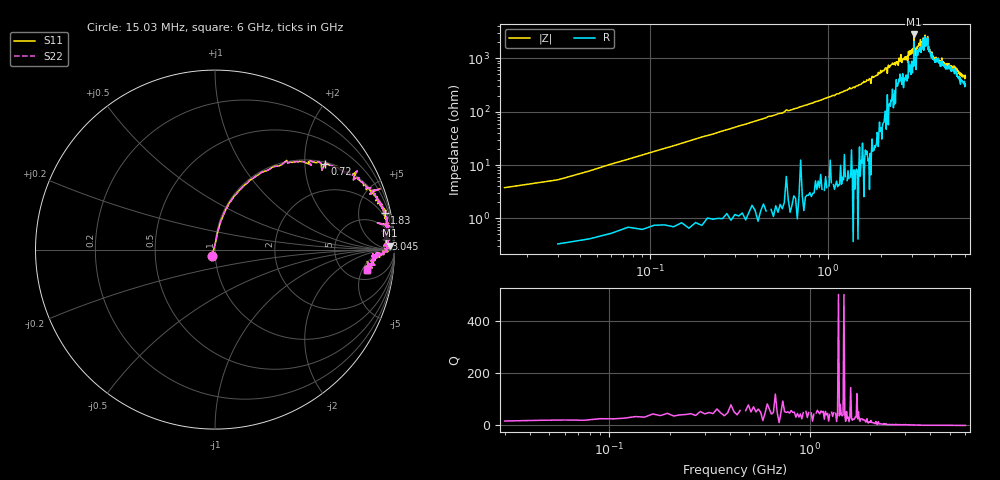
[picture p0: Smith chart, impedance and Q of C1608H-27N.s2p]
!	Network	Analyzer	HP8753E.07.74:	Oct	30	2002	Serial	No.	JP38451487
!	Hewlett-Packard
!	7	Sep	2009	10:22:24
!	Frequency	S11	S21	S12	S22
#	HZ	S	RI	R	50
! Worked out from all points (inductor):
!   400 points, 15.03 MHz to 6 GHz, reference 50 ohm
!   read as one part in series: L = 27.3 nH near 45.03 MHz
!   highest |Z| = 2.79 kohm at 3.075 GHz (marker M1)
!   self-resonance near 3.52 GHz
!   S11 on the Smith chart (normalised r, x): 15.03 MHz: 0.97, -0.07; 720 MHz: 1.05, +2.52; 1.83 GHz: 1.38, +9.08; 3.045 GHz: 15, +20; 6 GHz: 7.37, -6.16
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1.502992e7  -0.0162 -0.0339  1.02 0.0339  1.02 0.0339  -0.0162 -0.0339
9.002955e7  0.0291 0.149  0.971 -0.149  0.971 -0.149  0.0291 0.149
1.95029e8  0.106 0.297  0.894 -0.297  0.894 -0.297  0.106 0.297
7.200264e8  0.612 0.477  0.388 -0.477  0.388 -0.477  0.612 0.477
1.020025e9  0.775 0.407  0.225 -0.407  0.225 -0.407  0.775 0.407
1.830021e9  0.946 0.206  0.054 -0.206  0.054 -0.206  0.946 0.206
2.01002e9  0.952 0.172  0.0476 -0.172  0.0476 -0.172  0.952 0.172
2.595017e9  0.964 0.0741  0.0365 -0.0741  0.0365 -0.0741  0.964 0.0741
2.835016e9  0.936 0.0912  0.0645 -0.0912  0.0645 -0.0912  0.936 0.0912
2.865016e9  0.951 0.051  0.049 -0.051  0.049 -0.051  0.951 0.051
3.015015e9  0.973 0.0591  0.0266 -0.0591  0.0266 -0.0591  0.973 0.0591
3.045015e9  0.951 0.0602  0.0494 -0.0602  0.0494 -0.0602  0.951 0.0602
3.075015e9  0.973 0.0225  0.0266 -0.0225  0.0266 -0.0225  0.973 0.0225
3.090015e9  0.956 0.0476  0.044 -0.0476  0.044 -0.0476  0.956 0.0476
3.165014e9  0.947 0.0681  0.0529 -0.0681  0.0529 -0.0681  0.947 0.0681
3.555012e9  0.966 0.0113  0.0337 -0.0113  0.0337 -0.0113  0.966 0.0113
3.585012e9  0.945 0.00696  0.0553 -0.00696  0.0553 -0.00696  0.945 0.00696
3.675012e9  0.964 -0.0111  0.036 0.0111  0.036 0.0111  0.964 -0.0111
3.705011e9  0.936 -0.00909  0.0638 0.00909  0.0638 0.00909  0.936 -0.00909
4.00501e9  0.917 -0.0334  0.0826 0.0334  0.0826 0.0334  0.917 -0.0334
5.010005e9  0.883 -0.0521  0.117 0.0521  0.117 0.0521  0.883 -0.0521
6e9  0.845 -0.114  0.155 0.114  0.155 0.114  0.845 -0.114
